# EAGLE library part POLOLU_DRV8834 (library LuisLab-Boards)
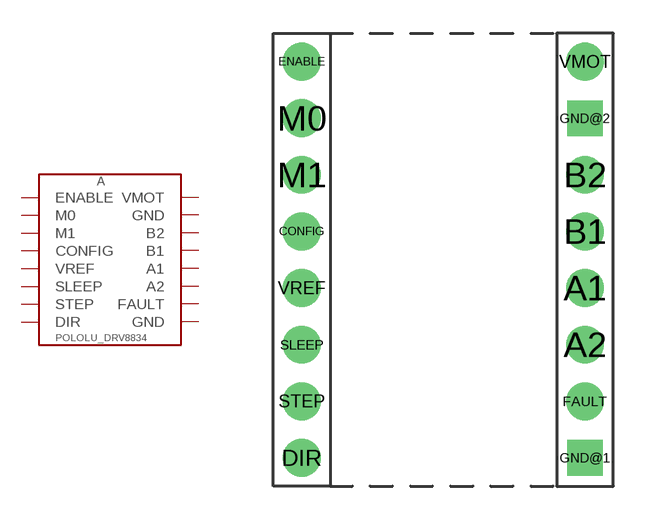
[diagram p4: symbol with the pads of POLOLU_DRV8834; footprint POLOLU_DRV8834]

Designator prefix A

## POLOLU_DRV8834  [POLOLU_DRV8834]
A1  A1
A2  A2
B1  B1
B2  B2
CONFIG  CONFIG
DIR  DIR
ENABLE  ENABLE
FAULT  FAULT
GND@1  GND
GND@2  GND
M0  M0
M1  M1
SLEEP  SLEEP
STEP  STEP
VMOT  VMOT
VREF  VREF

## Footprint POLOLU_DRV8834 (pad centres in mm)
drill 1.016 pad 1.7: A1 6.35,-1.27; A2 6.35,-3.81; B1 6.35,1.27; B2 6.35,3.81; CONFIG -6.35,1.27; DIR -6.35,-8.89; ENABLE -6.35,8.89; FAULT 6.35,-6.35; M0 -6.35,6.35; M1 -6.35,3.81; SLEEP -6.35,-3.81; STEP -6.35,-6.35; VMOT 6.35,8.89; VREF -6.35,-1.27
drill 1.016 pad 1.6 square: GND@1 6.35,-8.89; GND@2 6.35,6.35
